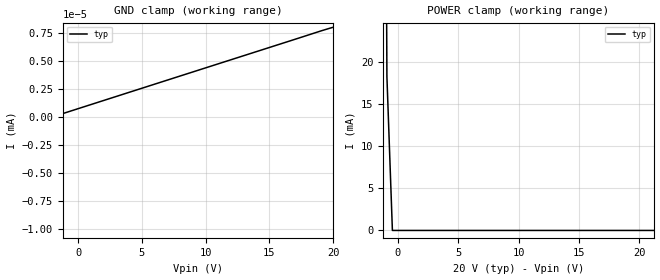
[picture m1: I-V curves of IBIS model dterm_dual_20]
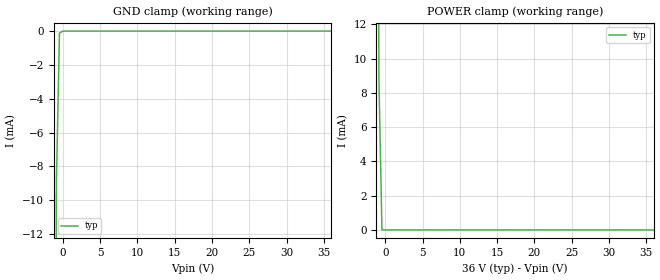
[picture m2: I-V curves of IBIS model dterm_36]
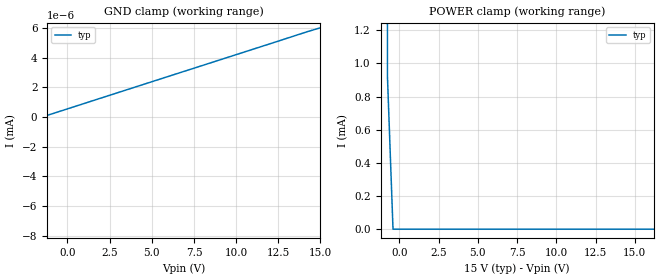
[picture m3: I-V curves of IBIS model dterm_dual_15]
|Texas Instruments Incorporated
|tmux7308f,  60V Fault-Protected, 8:1 Multiplexer with 1.8-V Logic
[IBIS Ver]   4.1
[File name]   tmux7308f.ibs
[Date]   12/08/21
[File Rev]   1.0
[Source]
| Texas Instruments Incorporated.
| ASC-INT-MPD
| 12500 TI Blvd
| Dallas, TX - 75243
[Notes]   Revision History:
| Rev 1.0: 12/08/21
| - Initial version of the model
| - Model generated from simulations in SPECTRE
| - C_comp although listed in numerical order of value are
|   obtained from varying PVT conditions. For PVT conditions for
|   each specific value refer the buffer description under
|   respective [Model]. IBIS model user is responsible for using
|   appropriate C_comp to simulate for Signal Integrity.
[Disclaimer]
| This model is designed as an aid for customers of Texas Instruments.
| TI and its licensors and suppliers make no warranties, either expressed
| or implied, with respect to this  model, including the warranties of
| merchantability or fitness for a particular purpose. The model is
| provided solely on an "as is" basis. The entire risk as to its quality
| and performance is with the customer.
| This model is subject to change without notice. Texas Instruments
| Incorporated is not responsible for updating this model.
[Copyright]
(C) Copyright 2021 Texas Instruments Incorporated.All rights reserved.
|  Component TMUX7308FPW 16-pin - PW package
|  Part # TMUX7308FPW
[Component]   TMUX7308FPW
[Manufacturer]  TI
[Package]
|   typ   min   max
R_pkg   0.0668   NA   NA
L_pkg   2.1992nH   NA   NA
C_pkg   0.2884pF   NA   NA
[Pin]   signal_name   model_name
   1   A0   inbuf
   2   EN   inbuf
   3   VSS   POWER
   4   S1   sterm
   5   S2   sterm
   6   S3   sterm
   7   S4   sterm
   8   D   dterm
   9   S8   sterm
   10   S7   sterm
   11   S6   sterm
   12   S5   sterm
   13   VDD   POWER
   14   GND   GND
   15   A2   inbuf
   16   A1   inbuf
[Series Switch Groups]
On 1 /
On 2 /
On 3 /
On 4 /
On 5 /
On 6 /
On 7 /
On 8 /
Off 1 2 3 4 5 6 7 8 /
[Series Pin Mapping]  pin_2 model_name function_table_group
   4   8   switch_dual_20   1
   5   8   switch_dual_20   2
   6   8   switch_dual_20   3
   7   8   switch_dual_20   4
  12   8   switch_dual_20   5
  11   8   switch_dual_20   6
  10   8   switch_dual_20   7
   9   8   switch_dual_20   8
|   4   8   switch_36   1
|   5   8   switch_36   2
|   6   8   switch_36   3
|   7   8   switch_36   4
|  12   8   switch_36   5
|  11   8   switch_36   6
|  10   8   switch_36   7
|   9   8   switch_36   8
|   4   8   switch_dual_15   1
|   5   8   switch_dual_15   2
|   6   8   switch_dual_15   3
|   7   8   switch_dual_15   4
|  12   8   switch_dual_15   5
|  11   8   switch_dual_15   6
|  10   8   switch_dual_15   7
|   9   8   switch_dual_15   8
|   4   8   switch_12   1
|   5   8   switch_12   2
|   6   8   switch_12   3
|   7   8   switch_12   4
|  12   8   switch_12   5
|  11   8   switch_12   6
|  10   8   switch_12   7
|   9   8   switch_12   8
|  Component TMUX7308FRRP 16-pin - RRP package
|  Part # TMUX7308FRRP
[Component]   TMUX7308FRRP
[Manufacturer]  TI
[Package]
|   typ   min   max
R_pkg   0.067   NA   NA
L_pkg   0.937nH   NA   NA
C_pkg   0.144pF   NA   NA
[Pin]   signal_name   model_name
   1   VSS   POWER
   2   S1   sterm
   3   S2   sterm
   4   S3   sterm
   5   S4   sterm
   6   D   dterm
   7   S8   sterm
   8   S7   sterm
   9   S6   sterm
   10   S5   sterm
   11   VDD   POWER
   12   GND   GND
   13   A2   inbuf
   14   A1   inbuf
   15   A0   inbuf
   16   EN   inbuf
[Series Switch Groups]
On 1 /
On 2 /
On 3 /
On 4 /
On 5 /
On 6 /
On 7 /
On 8 /
Off 1 2 3 4 5 6 7 8 /
[Series Pin Mapping]  pin_2 model_name function_table_group
   2   6   switch_dual_20   1
   3   6   switch_dual_20   2
   4   6   switch_dual_20   3
   5   6   switch_dual_20   4
  10   6   switch_dual_20   5
   9   6   switch_dual_20   6
   8   6   switch_dual_20   7
   7   6   switch_dual_20   8
|   2   6   switch_36   1
|   3   6   switch_36   2
|   4   6   switch_36   3
|   5   6   switch_36   4
|  10   6   switch_36   5
|   9   6   switch_36   6
|   8   6   switch_36   7
|   7   6   switch_36   8
|   2   6   switch_dual_15   1
|   3   6   switch_dual_15   2
|   4   6   switch_dual_15   3
|   5   6   switch_dual_15   4
|  10   6   switch_dual_15   5
|   9   6   switch_dual_15   6
|   8   6   switch_dual_15   7
|   7   6   switch_dual_15   8
|   2   6   switch_12   1
|   3   6   switch_12   2
|   4   6   switch_12   3
|   5   6   switch_12   4
|  10   6   switch_12   5
|   9   6   switch_12   6
|   8   6   switch_12   7
|   7   6   switch_12   8
[Model Selector] dterm
dterm_dual_20 Use for operation at +/-20V
dterm_36 Use for operation at 36V
dterm_dual_15 Use for operation at +/-15V
dterm_12 Use for operation at 12V
[Model Selector] sterm
sterm_dual_20 Use for operation at +/-20V
sterm_36 Use for operation at 36V
sterm_dual_15 Use for operation at +/-15V
sterm_12 Use for operation at 12V
[Model Selector] inbuf
inbuf_dual_20 Use for operation at +/-20V
inbuf_36 Use for operation at 36V
inbuf_dual_15 Use for operation at +/-15V
inbuf_12 Use for operation at 12V
| switch_dual_20
[Model]   switch_dual_20
Model_type   Series_switch
|   typ   min   max
C_comp   1.598234e-12   NA   NA
[Voltage Range]   20   NA   NA
[Power Clamp Reference]   20   NA   NA
[Temperature Range]   27   NA   NA
[On]
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[Off]
|   typ   min   max
[R Series]   10G   NA   NA
| switch_36
[Model]   switch_36
Model_type   Series_switch
|   typ   min   max
C_comp   1.598234e-12   NA   NA
[Voltage Range]   36   NA   NA
[Power Clamp Reference]   36   NA   NA
[Temperature Range]   27   NA   NA
[On]
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[Off]
|   typ   min   max
[R Series]   10G   NA   NA
| switch_dual_15
[Model]   switch_dual_15
Model_type   Series_switch
|   typ   min   max
C_comp   1.598234e-12   NA   NA
[Voltage Range]   15   NA   NA
[Power Clamp Reference]   15   NA   NA
[Temperature Range]   27   NA   NA
[On]
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[Off]
|   typ   min   max
[R Series]   10G   NA   NA
| switch_12
[Model]   switch_12
Model_type   Series_switch
|   typ   min   max
C_comp   2.533030e-12   NA   NA
[Voltage Range]   12   NA   NA
[Power Clamp Reference]   12   NA   NA
[Temperature Range]   27   NA   NA
[On]
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[Off]
|   typ   min   max
[R Series]   10G   NA   NA
| Models and submodels in the file (16): dterm_dual_20 (Terminator), dterm_36 (Terminator), dterm_dual_15 (Terminator), dterm_12 (Terminator), switch_dual_20 (Series_switch), switch_36 (Series_switch), switch_dual_15 (Series_switch), switch_12 (Series_switch), sterm_dual_20 (Terminator), sterm_36 (Terminator), sterm_dual_15 (Terminator), sterm_12 (Terminator), inbuf_dual_20 (Input), inbuf_36 (Input), inbuf_dual_15 (Input), inbuf_12 (Input)
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| dterm_dual_20
[Model]   dterm_dual_20
Model_type   Terminator
|   typ   min   max
C_comp   1.008417e-11   NA   NA
[Voltage Range]   20   NA   NA
[Temperature Range]   27   NA   NA
[Power Clamp Reference]   20   NA   NA
[GND Clamp Reference]   0   NA   NA
[GND Clamp]
|   Voltage   I(typ)   I(min)   I(max)
-25V      -1.414A    NA         NA
-20V      -5.041uA   NA         NA
-19.55V   -6.406nA   NA         NA
20V       8.043nA    NA         NA
[POWER Clamp]
|   Voltage   I(typ)   I(min)   I(max)
-5V       1.414A     NA         NA
-1.364V   155.3mA    NA         NA
-909.1mV  18.23mA    NA         NA
-454.5mV  68.57nA    NA         NA
40V       -5.036uA   NA         NA
| dterm_36
[Model]   dterm_36
Model_type   Terminator
|   typ   min   max
C_comp   1.008417e-11   NA   NA
[Voltage Range]   36   NA   NA
[Temperature Range]   27   NA   NA
[Power Clamp Reference]   36   NA   NA
[GND Clamp Reference]   0   NA   NA
[GND Clamp]
|   Voltage   I(typ)   I(min)   I(max)
-5V       -1.414A    NA         NA
-1.273V   -125.7mA   NA         NA
-858.6mV  -9.05mA    NA         NA
-444.4mV  -116uA     NA         NA
-30.3mV   -7.891uA   NA         NA
383.8mV   -5.778nA   NA         NA
36V       7.24nA     NA         NA
[POWER Clamp]
|   Voltage   I(typ)   I(min)   I(max)
-5V       1.414A     NA         NA
-1.273V   125.5mA    NA         NA
-858.6mV  8.924mA    NA         NA
-444.4mV  50.58nA    NA         NA
36V       -4.424uA   NA         NA
| dterm_dual_15
[Model]   dterm_dual_15
Model_type   Terminator
|   typ   min   max
C_comp   1.008417e-11   NA   NA
[Voltage Range]   15   NA   NA
[Temperature Range]   27   NA   NA
[Power Clamp Reference]   15   NA   NA
[GND Clamp Reference]   0   NA   NA
[GND Clamp]
|   Voltage   I(typ)   I(min)   I(max)
-20V      -1.414A    NA         NA
-15.05V   -11.62uA   NA         NA
-14.7V    -4.947nA   NA         NA
-14.34V   -4.692nA   NA         NA
15V       6.031nA    NA         NA
[POWER Clamp]
|   Voltage   I(typ)   I(min)   I(max)
-5V       1.414A     NA         NA
-1.111V   74.09mA    NA         NA
-757.6mV  919.6uA    NA         NA
-404mV    15.19nA    NA         NA
29.65V    -857.9pA   NA         NA
30V       -4.915uA   NA         NA
